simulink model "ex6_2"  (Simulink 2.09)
settings: Solver=FixedStepDiscrete  StartTime=0.0  StopTime=100.0  RelTol=1e-3  AbsTol=1e-6

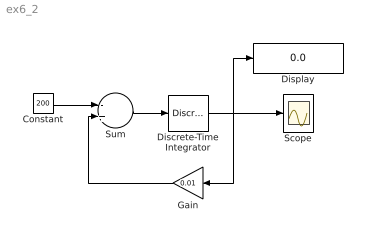
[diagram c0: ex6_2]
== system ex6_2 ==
  Constant : Constant  Value=200
  Discrete-Time Integrator : DiscreteIntegrator  IntegratorMethod=ForwardEuler  ExternalReset=none  InitialConditionSource=internal  InitialCondition=15000  LimitOutput=off  UpperSaturationLimit=inf  LowerSaturationLimit=-inf  ShowSaturationPort=off  ShowStatePort=off  SampleTime=1
  Display : Display
  Gain : Gain  Orientation=left  Gain=0.01
  Scope : Scope
  Sum : Sum  Inputs=-+
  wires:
  Sum/1 -> Discrete-Time Integrator/1
  Gain/1 -> Sum/2
  Constant/1 -> Sum/1
  Discrete-Time Integrator/1 -> Display/1, Scope/1, Gain/1
